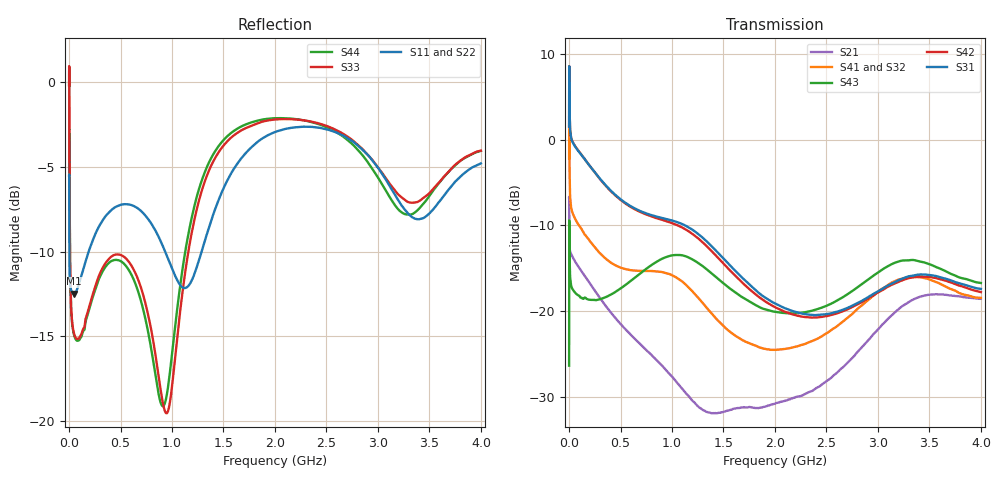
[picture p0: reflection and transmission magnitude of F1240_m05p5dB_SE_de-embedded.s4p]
! Integrated Device Technology
! Corporate Headquarters
! 6024 Silver Creek Valley Road
! San Jose, CA 95138  USA
! Phone:  1-408-284-8200
! Toll Free:  1-800-223-1366
! Webpage:  http://www.idt.com/
! Timing and RF Division
! 515 Groton Road, Suite 102
! Westford, MA 01886-6024
! Device:  F1240
! Description: Dual Intermediate Frequency Digital Variable Gain Amplifier
! Frequency:  10.0 -  500.00 MHz
! Package:  5x5 mm QFN Plastic Package: 32 pin
! Ports:  8 RF, 20 DC
!  Pin  1  = GA3 / Data  Pin 17  = RF OUT_B+
!  Pin  2  = GA4 / CLK  Pin 18  = RF OUT_B-
!  Pin  3  = GA5  Pin 19  = STBY_B
!  Pin  4  = VMODE  Pin 20  = Ground
!  Pin  5  = No Connect  Pin 21  = Ground
!  Pin  6  = GB5  Pin 22  = STB_A
!  Pin  7  = GB4  Pin 23  = RF OUT_A-  = Port 4
!  Pin  8  = GB3  Pin 24  = RF OUT_A+  = Port 3
!  Pin  9  = GB2  Pin 25  = GA0
!  Pin 10  = GB1  Pin 26  = ISET_A
!  Pin 11  = RF IN_B+  Pin 27  = VCC
!  Pin 12  = RF IN_B-  Pin 28  = Ground
!  Pin 13  = Ground  Pin 29  = RF IN_A-  = Port 2
!  Pin 14  = VCC  Pin 30  = RF IN_A+  = Port 1
!  Pin 15  = ISET_B  Pin 31  = GA1
!  Pin 16  = GB0  Pin 32  = GA2 / CSb
! Gain  = +19.5 dB
! State  = 1
! Voltage  = +5.00 V
! Current  = 85.292 mA (one channel only)
! Temperture  =  +25 C
! Test Date  =  2017-10-18
! Board  =  EB4031
! Data:  The device was measured on a custom evaluation board which has
!  individual transmission lines to the RF pins.  Data was collected
!  using a calibrated network analyzer.  The evaluation board was
!  de-embedded using Automatic Fixture Removal.
!  The reference plane is the edge of the package pin.
!  Only Channel A was measured.
!  This data is in single-ended operation.  If your needs are balanced
!  or differential S-parameters then this file needs to be used a
!  linear simulator.
! File Date:  2017-11-10  MJV
! Note:
!  Integrated Device Technology supplies this data as a sample of measured
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# Hz S dB R 100
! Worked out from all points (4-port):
!   410 points, 500 kHz to 4 GHz, reference 100 ohm
!   strongest paths, dB at 500 kHz, 930 MHz, 1.96 GHz, 2.98 GHz, 4 GHz:
!     S31: 1.5, -9.2, -18.8, -17.8, -17.4
!     S42: 1.5, -9.4, -19.3, -18.0, -17.8
!     S43: -26.3, -13.7, -20.0, -15.7, -16.7
!     S41: -2.2, -15.5, -24.5, -18.0, -18.4
!     S32: -2.1, -15.7, -24.4, -18.3, -18.8
!     S21: -6.7, -26.7, -30.9, -22.4, -18.6
!   lowest |S11| = -12.5 dB at 50 MHz (marker M1), VSWR 1.62, Z = 135 - j44.6 ohm
!   |S11| at or under -10 dB: 2.991 MHz to 190 MHz (187 MHz wide, 194 % of centre); 933.6 MHz to 1.287 GHz (353.5 MHz wide, 31.8 % of centre)
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500000  -5.51 -5.6  -6.70 -5.8  -31.25 78.6  -34.85 77.2
        -6.71 -5.9  -5.51 -5.6  -34.84 76.0  -31.24 79.7
        1.55 -109.8  -2.15 -112.0  -0.16 0.2  -26.33 -39.8
        -2.17 -110.9  1.55 -108.7  -26.34 -39.9  -0.17 2.5
2000000  -8.03 -30.3  -9.61 -30.7  -22.72 22.6  -27.07 6.0
         -9.62 -30.7  -8.01 -30.4  -27.03 5.7  -22.70 22.9
         7.96 177.9  3.57 161.4  -0.23 -53.4  -9.40 -144.4
         3.52 161.7  7.97 178.3  -9.40 -144.4  -0.27 -53.1
4000000  -10.90 -24.5  -12.34 -20.5  -23.45 5.4  -30.10 -11.8
         -12.35 -20.5  -10.90 -24.8  -30.05 -12.0  -23.44 5.6
         4.51 157.1  -2.15 139.6  -4.74 -86.8  -12.23 173.0
         -2.19 139.8  4.52 157.3  -12.23 172.9  -4.78 -86.7
5e7  -12.49 -41.0  -14.03 -23.9  -24.65 -16.8  -32.83 -19.4
     -14.03 -23.8  -12.45 -41.7  -32.83 -19.4  -24.61 -16.9
     -0.63 152.8  -9.02 142.0  -14.88 -162.2  -17.75 152.5
     -9.00 142.1  -0.58 152.6  -17.71 152.4  -14.96 -162.7
5.3e8  -7.20 -151.1  -21.89 -130.0  -27.97 -106.0  -36.26 -90.1
       -21.88 -129.8  -7.16 -152.1  -36.41 -88.0  -28.25 -106.1
       -7.22 24.2  -15.14 -30.8  -10.28 -175.2  -17.20 6.4
       -15.04 -32.2  -7.29 22.6  -17.10 6.0  -10.69 -175.8
2.9e9  -4.28 101.2  -23.49 -30.3  -27.73 -158.8  -30.00 -143.9
       -23.48 -30.4  -4.06 101.9  -30.66 -130.7  -29.14 -152.2
       -18.40 -73.7  -19.06 -156.4  -4.27 95.7  -17.18 -89.1
       -18.74 -168.0  -18.53 -70.4  -16.35 -87.3  -4.70 88.5
4e9  -4.79 -128.7  -18.56 116.2  -26.79 -32.6  -27.78 -17.2
     -18.56 116.1  -4.51 -127.5  -28.40 -2.8  -28.69 -23.8
     -17.40 45.4  -18.83 -52.2  -4.03 -133.4  -18.06 63.1
     -18.44 -66.5  -17.77 51.4  -16.71 56.0  -4.04 -143.2
